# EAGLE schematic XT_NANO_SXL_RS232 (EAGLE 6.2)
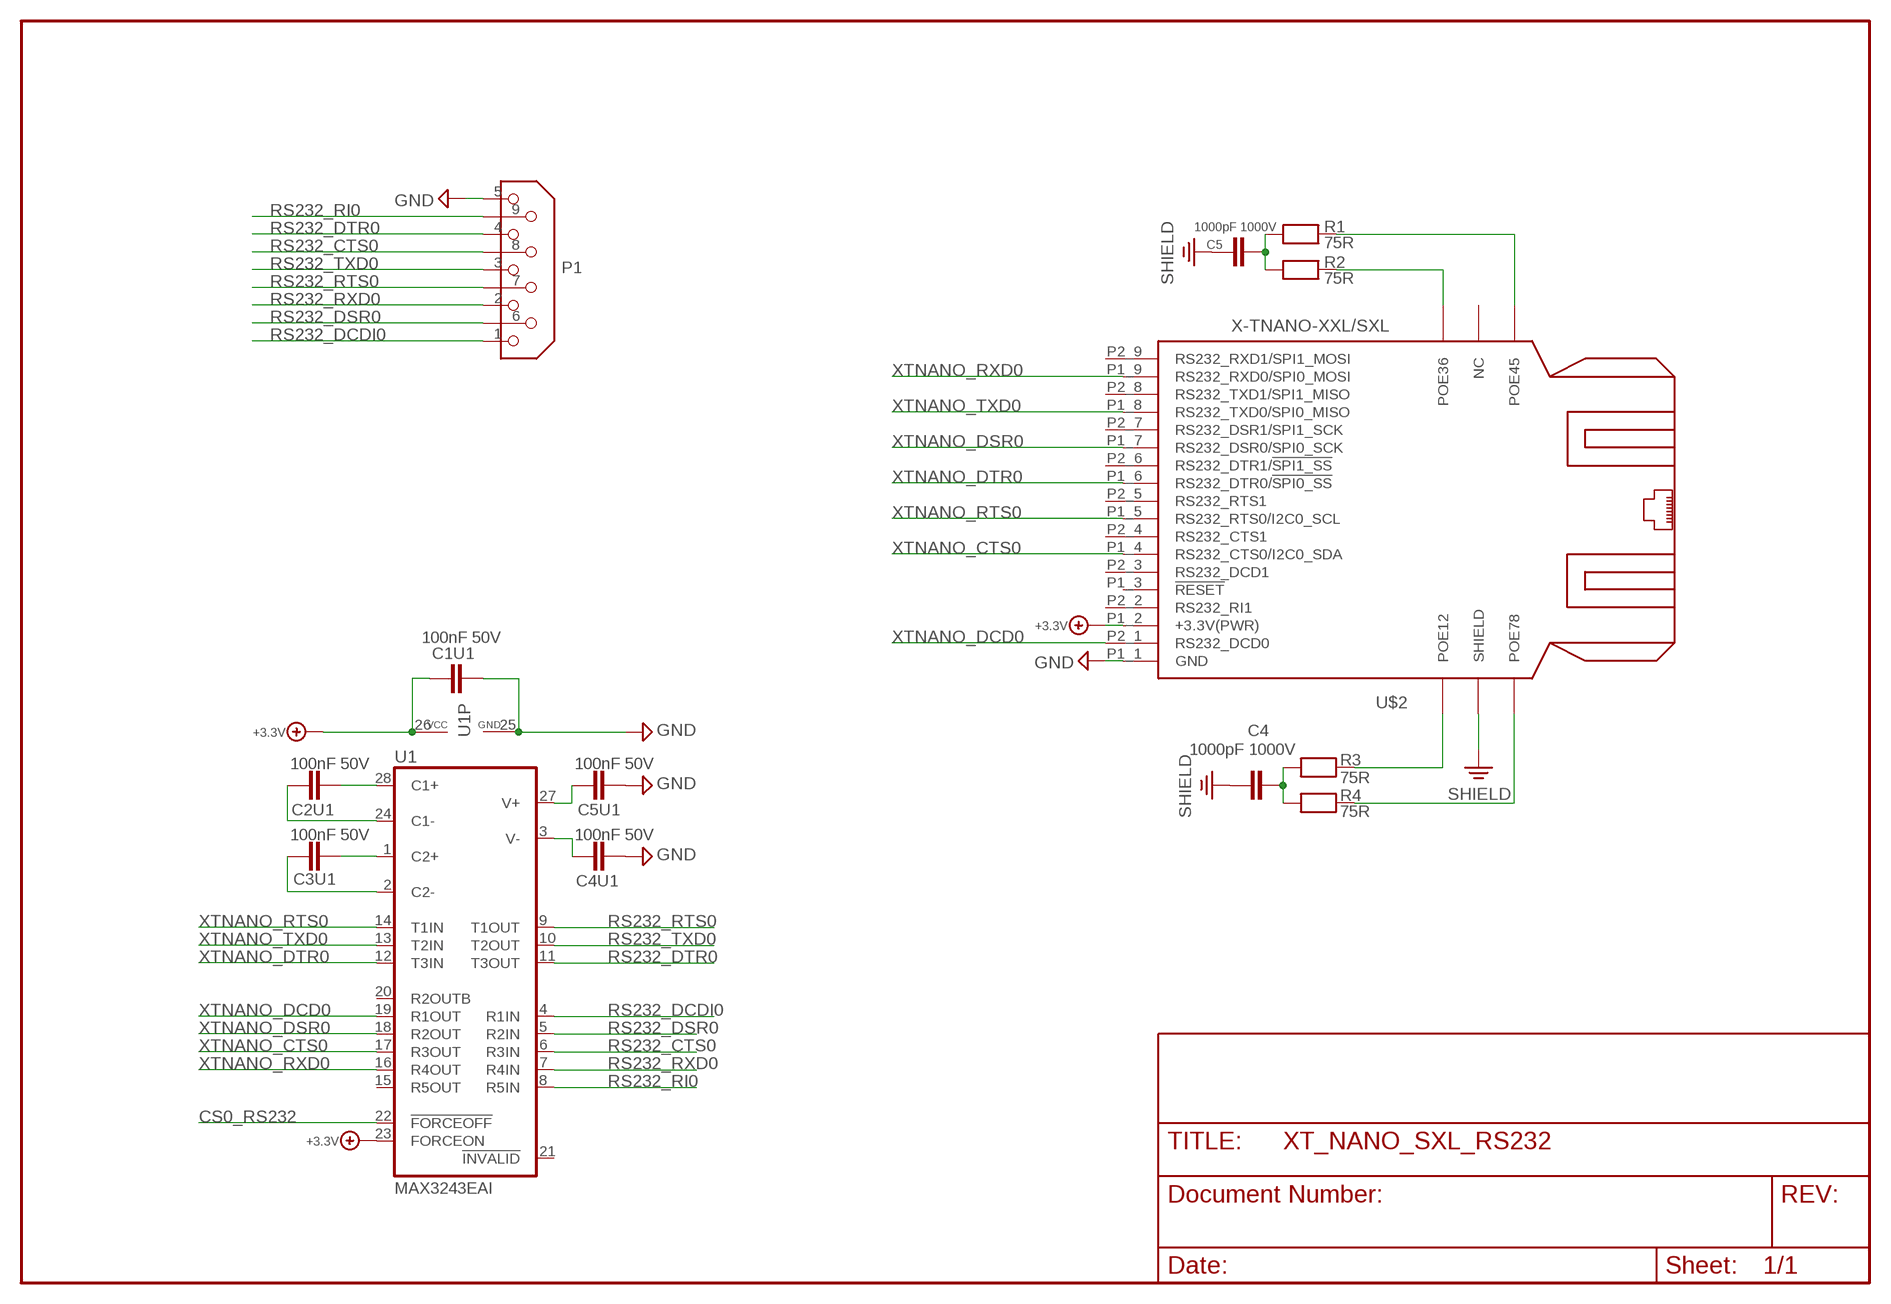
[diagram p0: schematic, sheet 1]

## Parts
C1U1  100nF 50V  CHIP-C-0603  [SMD-0603]
C2U1  100nF 50V  CHIP-C-0603  [SMD-0603]
C3U1  100nF 50V  CHIP-C-0603  [SMD-0603]
C4  1000pF 1000V  CHIP-C-1210  [SMD-1210]
C4U1  100nF 50V  CHIP-C-0603  [SMD-0603]
C5  1000pF 1000V  CHIP-C-1210  [SMD-1210]
C5U1  100nF 50V  CHIP-C-0603  [SMD-0603]
P1  DB9  [MSUB9-5]
R1  75R  CHIP-R-0603  [SMD-0603]
R2  75R  CHIP-R-0603  [SMD-0603]
R3  75R  CHIP-R-0603  [SMD-0603]
R4  75R  CHIP-R-0603  [SMD-0603]
U1  MAX3243EAI  [SSOP28]
U$2  X-TNANO-XXL/SXL  [XT-NANO-XXL/SXL]

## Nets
+3.3V: C1U1.1 U1.23(FORCEON) U1.26(VCC) U$2.P1_2(+3.3V(PWR))
CS0_RS232: U1.22(!FORCEOFF)
GND: C1U1.2 C4U1.2 C5U1.2 P1.5 U1.25(GND) U$2.P1_1(GND)
N$1: C5.1 R1.1 R2.1
N$2: C4.2 R3.1 R4.1
N$4: R2.2 U$2.POE36
N$6: R1.2 U$2.POE45
N$20: R3.2 U$2.POE12
N$21: R4.2 U$2.POE78
N$22: C4U1.1 U1.3(V-)
N$23: C5U1.1 U1.27(V+)
N$24: C3U1.2 U1.1(C2+)
N$26: C2U1.2 U1.28(C1+)
N$27: C3U1.1 U1.2(C2-)
N$28: C2U1.1 U1.24(C1-)
RS232_CTS0: P1.8 U1.6(R3IN)
RS232_DCDI0: P1.1 U1.4(R1IN)
RS232_DSR0: P1.6 U1.5(R2IN)
RS232_DTR0: P1.4 U1.11(T3OUT)
RS232_RI0: P1.9 U1.8(R5IN)
RS232_RTS0: P1.7 U1.9(T1OUT)
RS232_RXD0: P1.2 U1.7(R4IN)
RS232_TXD0: P1.3 U1.10(T2OUT)
SHIELD: C4.1 C5.2 U$2.SHIELD
XTNANO_CTS0: U1.17(R3OUT) U$2.P1_4(RS232_CTS0/I2C0_SDA)
XTNANO_DCD0: U1.19(R1OUT) U$2.P2_1(RS232_DCD0)
XTNANO_DSR0: U1.18(R2OUT) U$2.P1_7(RS232_DSR0/SPI0_SCK)
XTNANO_DTR0: U1.12(T3IN) U$2.P1_6(RS232_DTR0/!SPI0_SS!)
XTNANO_RTS0: U1.14(T1IN) U$2.P1_5(RS232_RTS0/I2C0_SCL)
XTNANO_RXD0: U1.16(R4OUT) U$2.P1_9(RS232_RXD0/SPI0_MOSI)
XTNANO_TXD0: U1.13(T2IN) U$2.P1_8(RS232_TXD0/SPI0_MISO)
Unconnected: U1.15(R5OUT) U1.20(R2OUTB) U1.21(!INVALID) U$2.FLASH(NC) U$2.P1_3(!RESET) U$2.P2_2(RS232_RI1) U$2.P2_3(RS232_DCD1) U$2.P2_4(RS232_CTS1) U$2.P2_5(RS232_RTS1) U$2.P2_6(RS232_DTR1/!SPI1_SS!) U$2.P2_7(RS232_DSR1/SPI1_SCK) U$2.P2_8(RS232_TXD1/SPI1_MISO) U$2.P2_9(RS232_RXD1/SPI1_MOSI)

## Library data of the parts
C1U1 C2U1 C3U1 C4U1 C5U1 = mea-lib:CHIP-C-?: Chip capacitance
C4 C5 = XTMACRO:CHIP-C-?: Chip capacitance
P1 = XTMACRO:DB9
R1-R4 = XTMACRO:CHIP-R-?: Chip resistors
U1 = maxim:MAX3243*: RS-232 Transceivers with AutoShutdown 1µA Supply-Current, True +3V to +5.5V http://dbserv.maxim-ic.com/
U$2 = ak-devices:X-TNANO-XXL/SXL: AK-NORD XT-NANO-XXL/SXL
